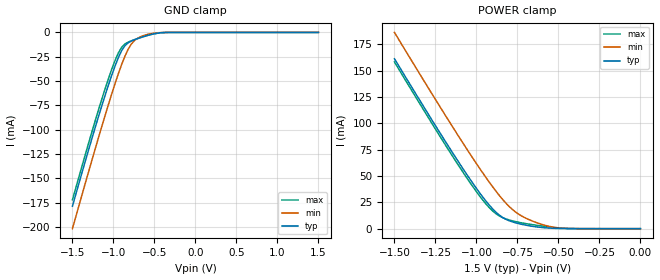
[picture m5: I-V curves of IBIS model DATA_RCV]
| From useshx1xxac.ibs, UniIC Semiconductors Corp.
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|   Model DATA_RCV
[Model]  DATA_RCV
Model_type   Input
Polarity   Non-Inverting
Vinl =   0.600000V
Vinh =   0.900000V
C_comp   1.3900pF   1.3640pF   1.5600pF
[Temperature Range]   25.0000   95.0000   0.0
[Voltage Range]   1.5000V   1.4000V   1.6000V
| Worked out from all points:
|   GND clamp passes 1 mA (typ) near -0.48 V on its own axis
|   POWER clamp passes 1 mA (typ) near -0.59 V on its own axis
[GND_clamp]
|Voltage   I(typ)   I(min)   I(max)
-1.5V     -178.7mA   -201.8mA   -172.1mA
-1.18V    -85.9mA    -107.5mA   -79.02mA
-1.06V    -53.85mA   -73.82mA   -47.38mA
-980mV    -34.46mA   -52.52mA   -28.79mA
-940mV    -25.94mA   -42.47mA   -21.09mA
-900mV    -18.8mA    -33.04mA   -15.34mA
-860mV    -13.68mA   -24.5mA    -11.91mA
-780mV    -8.804mA   -11.75mA   -8.617mA
-740mV    -7.413mA   -8.071mA   -7.384mA
-620mV    -3.934mA   -2.917mA   -4.046mA
-420mV    -302.4uA   -187.9uA   -428.5uA
1.5V      1.623nA    17.64nA    1.98nA
[POWER_clamp]
|Voltage   I(typ)   I(min)   I(max)
-1.5V     161.3mA    186.3mA    158.3mA
-1.22V    90.37mA    115.2mA    87.1mA
-1.04V    47.2mA     71.18mA    43.94mA
-980mV    33.96mA    57.17mA    30.91mA
-920mV    22.07mA    43.79mA    19.67mA
-880mV    15.49mA    35.42mA    14.07mA
-840mV    10.61mA    27.72mA    10.46mA
-780mV    6.409mA    18.15mA    7.405mA
-720mV    3.991mA    11.66mA    5.381mA
-560mV    586.1uA    2.318mA    1.645mA
-440mV    47uA       184.9uA    218uA
0V        1.623nA    5.301nA    2.263nA
